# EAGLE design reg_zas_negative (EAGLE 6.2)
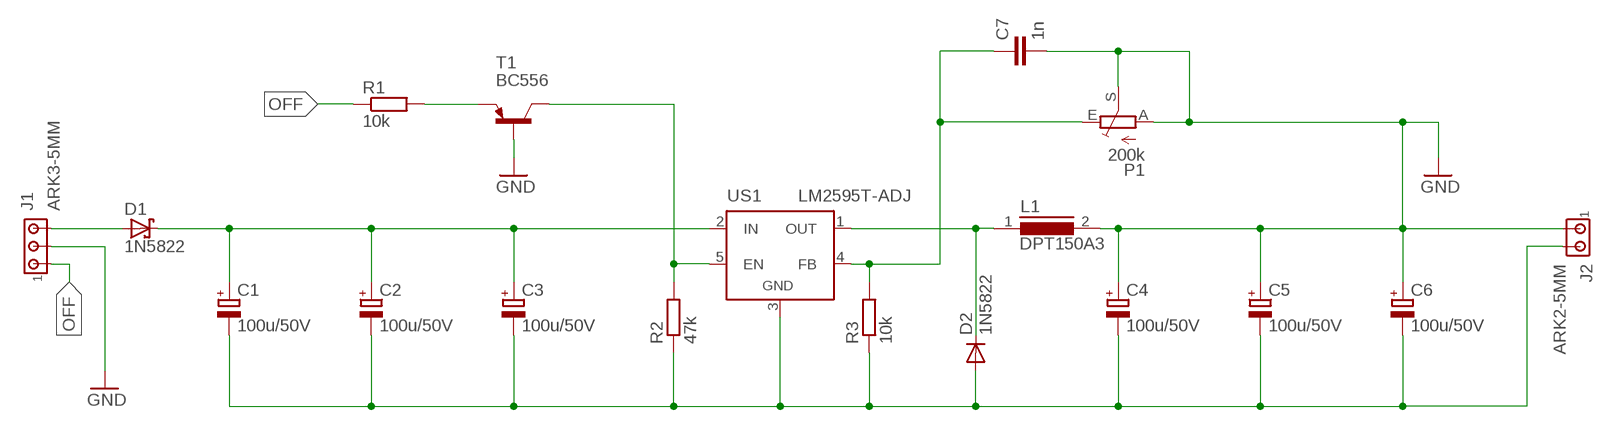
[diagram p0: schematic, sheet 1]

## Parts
C1  100u/50V  CPOL-EUE5-10.5  [E5-10,5]
C2  100u/50V  CPOL-EUE5-10.5  [E5-10,5]
C3  100u/50V  CPOL-EUE5-10.5  [E5-10,5]
C4  100u/50V  CPOL-EUE5-10.5  [E5-10,5]
C5  100u/50V  CPOL-EUE5-10.5  [E5-10,5]
C6  100u/50V  CPOL-EUE5-10.5  [E5-10,5]
C7  1n  C-EU050-025X075  [C050-025X075]
D1  1N5822  SCHOTTKY-DIODECB429-17  [CB429-17]
D2  1N5822  DIODE-SOD64-10  [SOD64-10]
J1  ARK3-5MM  [3PIN-5MM]
J2  ARK2-5MM  [2PIN-5MM]
L1  DPT150A3  SFT830D  [SFT830D]
P1  200k  TRIM_EU-B64Y  [B64Y]
R1  10k  R-EU_0207/7  [0207/7]
R2  47k  R-EU_0207/7  [0207/7]
R3  10k  R-EU_0207/7  [0207/7]
T1  BC556  [TO92-EBC]
US1  LM2595T-ADJ  LM2595TV  [TO220-51]

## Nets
GND: C4.+ C5.+ C6.+ C7.2 J1.P$2 J2.P$1 L1.2 P1.A P1.S T1.B
N$1: D1.A J1.P$3
N$2: C1.+ C2.+ C3.+ D1.C US1.2(IN)
N$3: R2.2 T1.C US1.5(EN)
N$4: R1.2 T1.E
N$5: C1.- C2.- C3.- C4.- C5.- C6.- D2.A J2.P$2 R2.1 R3.1 US1.3(GND)
N$6: D2.C L1.1 US1.1(OUT)
N$10: C7.1 P1.E R3.2 US1.4(FB)
OFF: J1.P$1 R1.1

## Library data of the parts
C1-C6 = rcl:CPOL-EU: POLARIZED CAPACITOR, European symbol
C7 = rcl:C-EU: CAPACITOR, European symbol
D1 = diode:SCHOTTKY-DIODE: Schottky Diode
D2 = diode:DIODE-: DIODE
J1 = zlacza_futrzak:ARK3: ARK 3 Raster 5mm i 3,5mm
J2 = zlacza_futrzak:ARK2: ARK 2
L1 = inductors:SFT830D: INDUCTOR
P1 = pot:TRIM_EU-: POTENTIOMETER
R1-R3 = rcl:R-EU_: RESISTOR, European symbol
T1 = transistor-pnp:BC556*: PNP Transistror
US1 = scalaki_futrzak:LM2595T: STEP-DOWN VOLTAGE REGULATOR

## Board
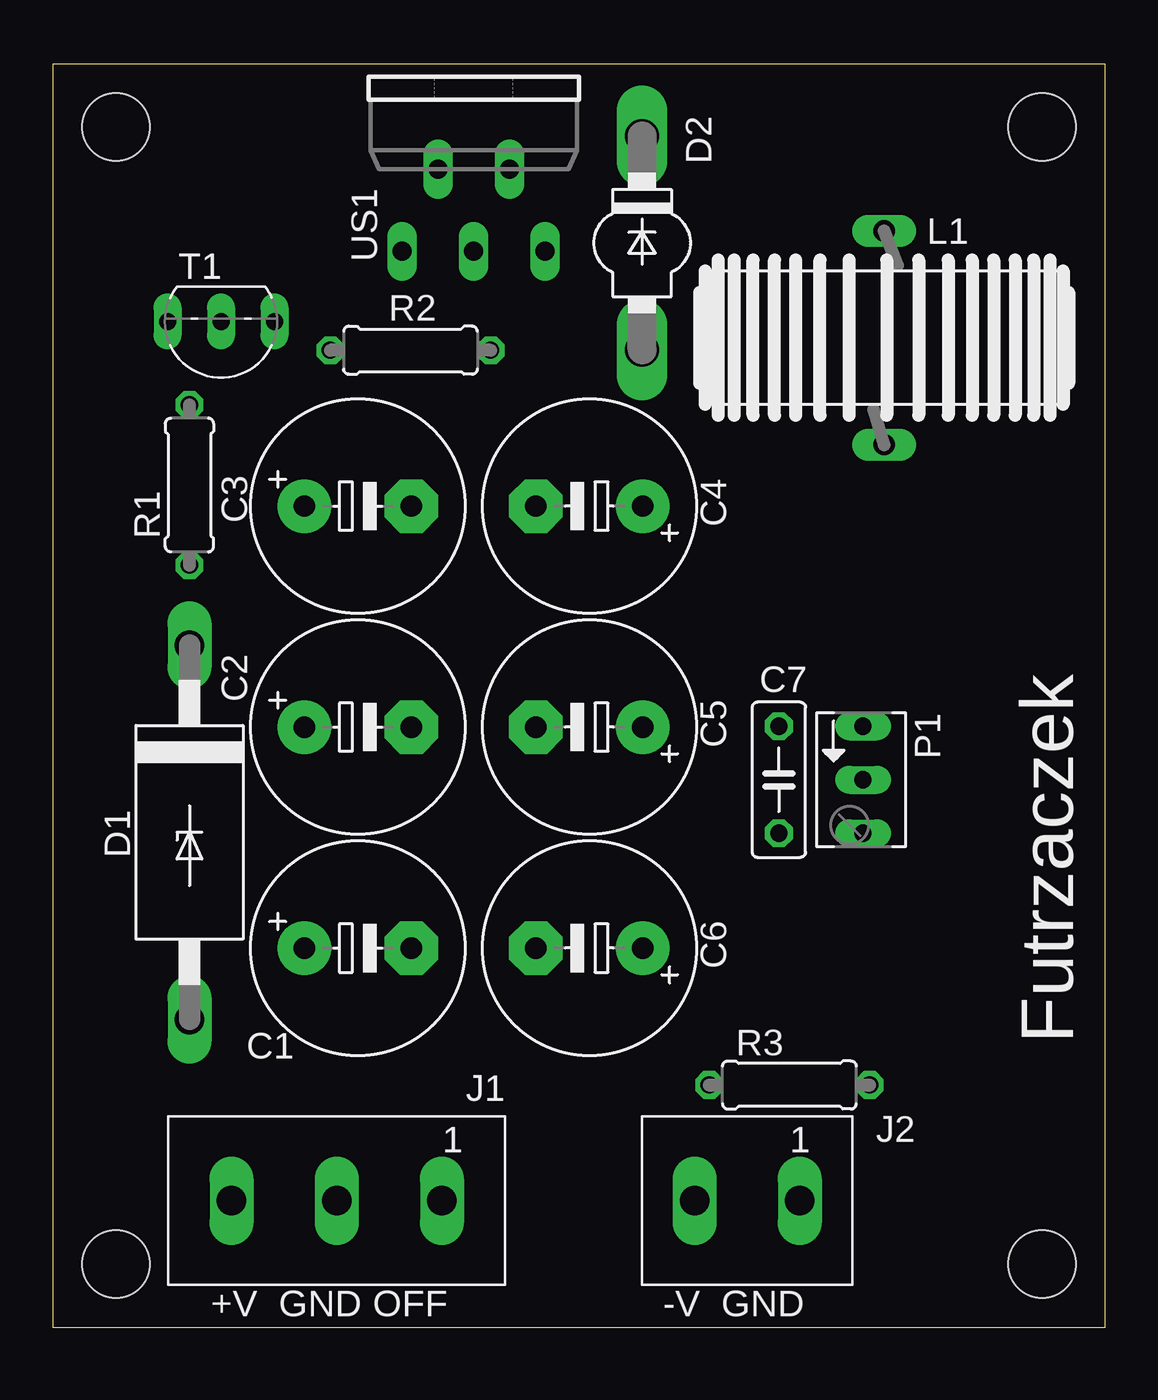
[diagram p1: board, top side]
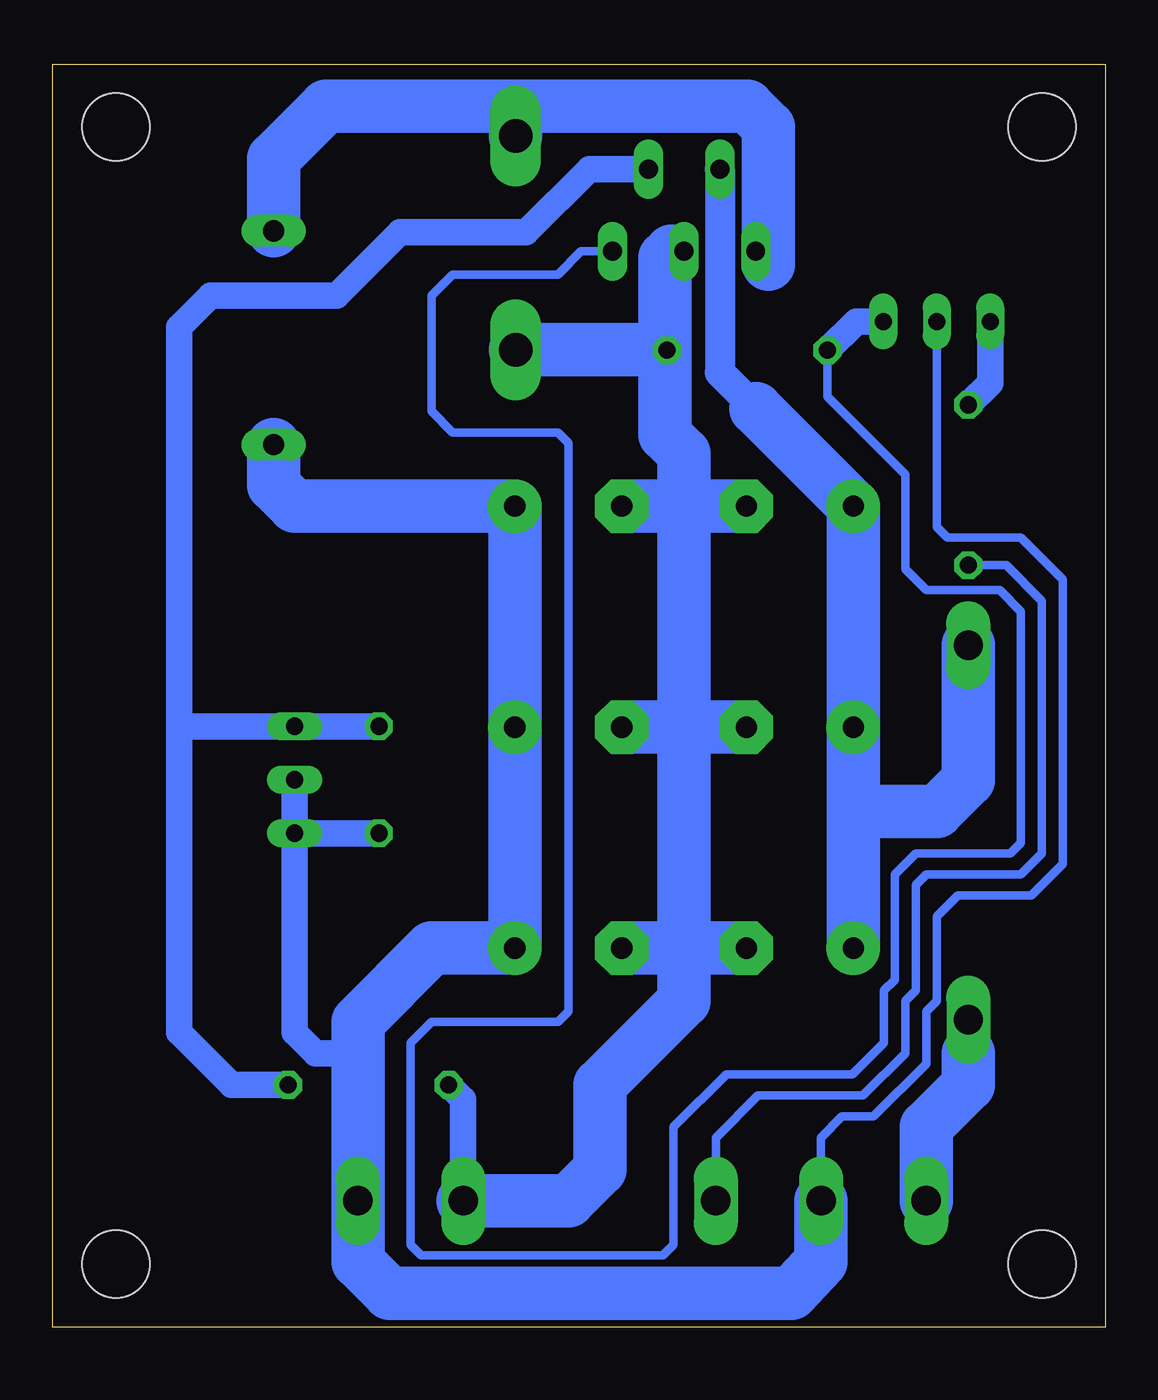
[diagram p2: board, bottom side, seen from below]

Size 50 x 60 mm. Coordinates in mm from the lower left corner, seen from the top.
Outline: 0,0 50,0 50,60 0,60 0,0
Copper layers (1*16): Top 0.035mm / dielectric 1.5mm / Bottom 0.035mm
Design rules: minimum track width 10mil, minimum drill 24mil, track to track 8mil, track to pad 8mil, pad to pad 8mil, via to via 8mil, smd to smd 8mil, copper to edge 10mil, drill to drill 8mil, minimum pad ring 10mil, minimum via ring 8mil, stop-mask expansion 4mil, vias tented up to drill 0mil, thermal gap 10mil
Holes 3.2 mm at 3,3 3,57 47,3 47,57

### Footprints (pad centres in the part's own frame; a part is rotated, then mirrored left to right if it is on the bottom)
E5-10,5 = drill 1.016 pad 2.54: + -2.54,0 | drill 1.016 pad 2.54 octagon: - 2.54,0
C050-025X075 = drill 0.813 octagon: 1 -2.54,0; 2 2.54,0
CB429-17 = drill 1.397 long: A 8.89,0; C -8.89,0
SOD64-10 = drill 1.6 long: A 5.08,0; C -5.08,0
3PIN-5MM = drill 1.4 long: P$1 -5,0; P$2 0,0; P$3 5,0
2PIN-5MM = drill 1.4 long: P$1 -2.5,0; P$2 2.5,0
SFT830D = drill 1.016 long: 1 -5.08,0; 2 5.08,0
B64Y = drill 0.813 long: A 2.54,0; E -2.54,0; S 0,0
0207/7 = drill 0.813 octagon: 1 -3.81,0; 2 3.81,0
TO92-EBC = drill 0.813 long: B 0,-1.27; C -2.54,-1.27; E 2.54,-1.27
TO220-51 = drill 0.9 long: 1 -3.4,-8.4; 2 -1.7,-4.5; 3 0,-8.4; 4 1.7,-4.5; 5 3.4,-8.4

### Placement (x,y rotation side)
C1  14.5,18 0 top
C2  14.5,28.5 0 top
C3  14.5,39 0 top
C4  25.5,39 180 top
C5  25.5,28.5 180 top
C6  25.5,18 180 top
C7  34.5,26 270 top
D1  6.5,23.5 270 top
D2  28,51.5 270 top
J1  13.5,6 180 top
J2  33,6 180 top
L1  39.5,47 270 top
P1  38.5,26 270 top
R1  6.5,40 90 top
R2  17,46.4 180 top
R3  35,11.5 0 top
T1  8,46.5 180 top
US1  20,59.5 0 top

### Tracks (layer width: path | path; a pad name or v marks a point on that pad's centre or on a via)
GND
  Bottom 0.406: T1.B 8,38 7.5,37.5 4,37.5 2,35.5 2,22 3.5,20.5 7,20.5 8,19.5 8,15.5 8.5,15 8.5,12.5 11,10 12.5,10 13.5,9 J1.P$2
  Bottom 1.27: P1.S P1.A | P1.A 38.5,14 37.5,13 35.5,13 | C7.2 P1.A
  Bottom 2.54: J1.P$2 13.5,3.1 14.9,1.6 34,1.6 35.5,3.1 J2.P$1 35.5,13 35.5,14.5 32,18 C6.+ C5.+ C4.+ 38.5,39 39.5,40 L1.2
N$1
  Bottom 1.778: 6.5,13 D1.A
  Bottom 2.54: J1.P$3 8.5,9.5 6.5,11.5 6.5,13
N$2
  Bottom 1.422: US1.2 18.3,45.34 16.6,43.64
  Bottom 2.54: 16.6,43.64 C3.+ C2.+ 11.96,24.5 | 11.96,24.5 C1.+ | D1.C 6.5,26 8,24.5 11.96,24.5
N$3
  Bottom 0.406: US1.5 24.9,51.1 26,50 31,50 32,49 32,43.5 31,42.5 26,42.5 25.5,42 25.5,15 26,14.5 32,14.5 33,13.5 33,3.9 32.5,3.4 21,3.4 20.5,3.9 20.5,9.5 18,12 12,12 10.5,13.5 10.5,16 10,16.5 10,21.5 9,22.5 4.5,22.5 4,23 4,34 5,35 8.5,35 9.5,36 9.5,40.5 13.19,44.19 R2.2
  Bottom 1.27: T1.C 11.82,47.77 R2.2
N$4
  Bottom 1.27: T1.E 5.46,44.85 R1.2
N$5
  Bottom 1.27: J2.P$2 30.5,10.81 R3.1 | 20.6,51.1 US1.3
  Bottom 1.778: 21.4,46.3 20.91,46.3 R2.1 20.81,46.09 20.9,46
  Bottom 2.54: C1.- 20,18 | C2.- 20,28.5 | C3.- 20,39 | 20,39 20,28.5 | 20,28.5 20,18 | C5.- 20,28.5 | C4.- 20,39 | 20,39 20,41.5 20.9,42.4 20.9,46 20.9,50.8 20.6,51.1 | D2.A 21.52,46.42 21.4,46.3 | 20,18 20,15.5 24,11.5 24,7.5 25.5,6 J2.P$2 | C6.- 20,18
N$6
  Bottom 1.27: 16,50.5 US1.1
  Bottom 2.54: 28,58 17,58 16,57 16,50.5 | 28,58 37,58 39.5,55.5 L1.1 | D2.C 28,58
N$10
  Bottom 1.27: R3.2 41.5,11.5 44,14 44,28.5 | 44,28.5 44,47.5 42.5,49 36.5,49 33.5,52 27.5,52 24.5,55 US1.4 | C7.1 P1.E 43.96,28.54 44,28.5
OFF
  Bottom 0.406: R1.1 4.69,36.19 3,34.5 3,22.5 4,21.5 8.5,21.5 9,21 9,16 9.5,15.5 9.5,13 11.5,11 16.5,11 18.5,9 J1.P$1

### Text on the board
tPlace: Futrzaczek | +V GND OFF | -V GND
